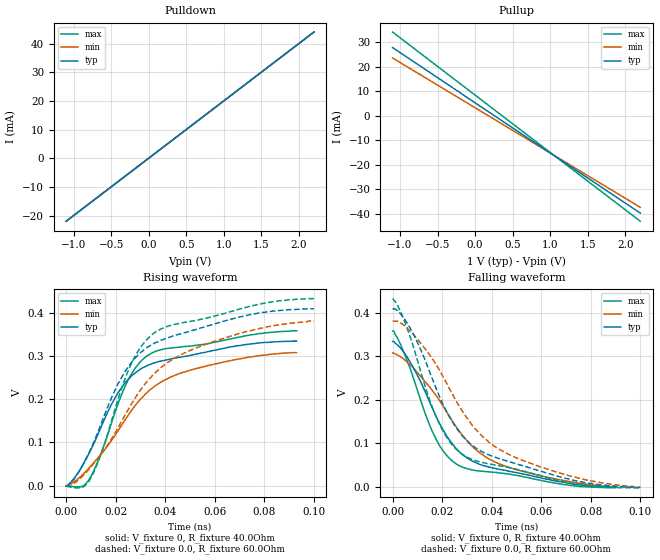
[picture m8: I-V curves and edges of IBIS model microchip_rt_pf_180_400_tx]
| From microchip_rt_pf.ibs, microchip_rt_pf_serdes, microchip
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[Model]   microchip_rt_pf_180_400_tx
Model_type   Output
Polarity   Non-Inverting
Enable   Active-High
Vmeas = 0.5
|   typ   min   max
C_comp   0.407p  0.407p  0.407p
[Voltage Range]   1.0  0.9  1.1
[Temperature Range]   27  27  27
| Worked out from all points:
|   slope of the pulldown table from 0 to 0.15 V, typ, clamps not added: 50 ohm
|   slope of the pullup table from 0 to 0.15 V, typ, clamps not added: 48.8 ohm
|   rising waveform, V_fixture 0, R_fixture 40.0Ohm: 20-80 % time 20.9ps typ, 28ps min, 16.1ps max; typ from 0 V to 0.334 V
|   rising waveform, V_fixture 0.0, R_fixture 60.0Ohm: 20-80 % time 25.3ps typ, 32.5ps min, 19.1ps max; typ from -0.001 V to 0.41 V
|   falling waveform, V_fixture 0, R_fixture 40.0Ohm: 20-80 % time 21.2ps typ, 27.4ps min, 16ps max; typ from 0.334 V to -0.001 V
|   falling waveform, V_fixture 0.0, R_fixture 60.0Ohm: 20-80 % time 25.7ps typ, 31.8ps min, 19ps max; typ from 0.41 V to -0.001 V
[Pullup]
|   X   TYP   MIN   MAX
-1.1V     27.83mA    23.59mA    34.19mA
1.01V     -15.43mA   -15.43mA   -15.26mA
1.066V    -16.58mA   -16.47mA   -16.57mA
2.2V      -39.82mA   -37.44mA   -43.14mA
[Pulldown]
|   X   TYP   MIN   MAX
-1.1V     -21.95mA   -21.98mA   -21.92mA
1.01V     20.22mA    20.21mA    20.23mA
1.089V    21.79mA    21.78mA    21.8mA
2.2V      44mA       44mA       44mA
[Ramp]
R_load = 50.0Ohm
|   typ   min   max
dV/dt_r   2.01E-1V/2.09E-2ns   1.85E-1V/2.80E-2ns   2.16E-1V/1.61E-2ns
dV/dt_f   2.01E-1V/2.12E-2ns   1.85E-1V/2.74E-2ns   2.16E-1V/1.60E-2ns
[Rising Waveform]
V_fixture   = 0
V_fixture_min = 0
V_fixture_max = 0
R_fixture   = 40.0Ohm
|   Time   V(typ)   V(min)   V(max)
0s        -500uV     -500uV     -1mV
6ps       41.15mV    22.19mV    -2.499mV
9ps       72.7mV     39.23mV    11.88mV
18ps      185.1mV    102.4mV    140.1mV
24ps      239.7mV    154.5mV    232.9mV
28ps      261.7mV    186.6mV    273.3mV
33ps      279mV      217.5mV    301.7mV
42ps      292.7mV    251.1mV    318.7mV
55ps      307.5mV    274.9mV    326.6mV
93ps      334.5mV    308mV      358.5mV
[Rising Waveform]
V_fixture   = 0.0
V_fixture_min = 0.0
V_fixture_max = 0.0
R_fixture   = 60.0Ohm
|   Time   V(typ)   V(min)   V(max)
0s        -1mV       -1mV       -1.5mV
6ps       40.77mV    18.73mV    -4.522mV
10ps      85.68mV    43.69mV    18.52mV
14ps      141.8mV    72.3mV     72.43mV
19ps      212.7mV    115mV      163.8mV
26ps      282.8mV    185.9mV    279mV
35ps      327.8mV    256mV      351.5mV
44ps      347.7mV    296.1mV    373.7mV
60ps      374.8mV    334.7mV    392.8mV
100ps     409.5mV    381mV      433mV
[Falling Waveform]
V_fixture   = 0
V_fixture_min = 0
V_fixture_max = 0
R_fixture   = 40.0Ohm
|   Time   V(typ)   V(min)   V(max)
0s        334.5mV    308mV      358.5mV
3ps       320.9mV    299.8mV    330.5mV
8ps       278.3mV    276.1mV    257.6mV
17ps      169.5mV    214.7mV    116.3mV
21ps      125.1mV    180.3mV    78.52mV
26ps      86.37mV    135.8mV    51.84mV
33ps      57.4mV     88.79mV    38.23mV
43ps      40.63mV    53.16mV    32.2mV
66ps      13.73mV    18.07mV    8.566mV
90ps      -1mV       0V         -1.5mV
[Falling Waveform]
V_fixture   = 0.0
V_fixture_min = 0.0
V_fixture_max = 0.0
R_fixture   = 60.0Ohm
|   Time   V(typ)   V(min)   V(max)
0s        409.5mV    381mV      433mV
4ps       392.1mV    374.2mV    392.8mV
8ps       355.8mV    353.4mV    329.8mV
18ps      220.9mV    277.6mV    155.9mV
23ps      160.6mV    225.5mV    104.4mV
28ps      118.5mV    175.8mV    75.67mV
37ps      78.47mV    112.4mV    55.47mV
48ps      56.42mV    71.65mV    43.37mV
74ps      14.38mV    21.99mV    6.579mV
100ps     -1mV       -494.8uV   -2mV
[Algorithmic Model]
Executable Linux_gcc5.4_64   MPF300T-TX_LX64.so   MPF300T-TX-R180_400.ami
Executable Windows_cl18.00.40629_64 MPF300T-TX_WIN64.dll  MPF300T-TX-R180_400.ami
Executable Windows_cl18.00.40629_32 MPF300T-TX_WIN32.dll  MPF300T-TX-R180_400.ami
[End Algorithmic Model]
